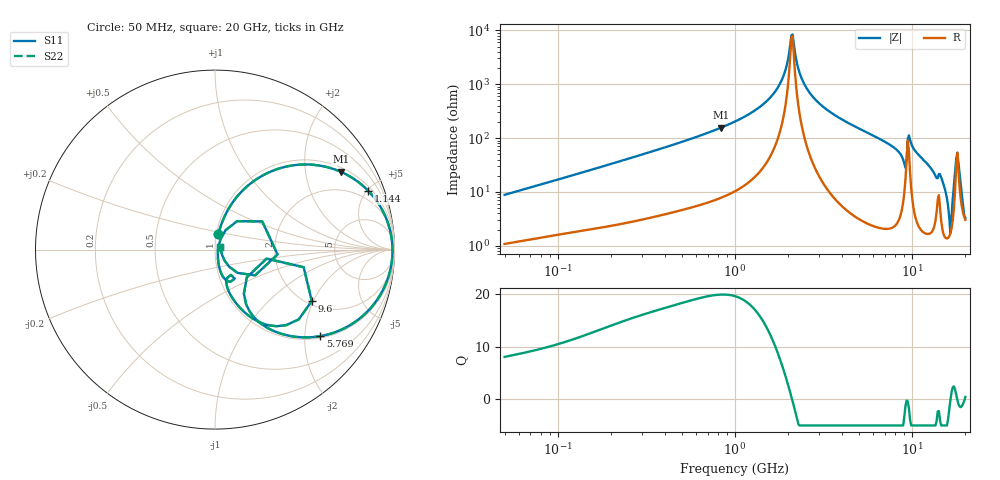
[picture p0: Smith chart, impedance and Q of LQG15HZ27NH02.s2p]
!Murata Part Number: LQG15HZ27NH02
!These Parameters are Measured in Series Mode Connection
!  o--[Z]--o
!Port1  Port2
!  o-------o
!Freq. Start=50[MHz] Stop=20[GHz], 401[Steps]
# Hz S RI R 50
!Freq.(Hz) S11(Real) S11(Imag) S21(Real) S21(Imag) S12(Real) S12(Imag) S22(Real) S22(Imag)
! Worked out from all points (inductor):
!   401 points, 50 MHz to 20 GHz, reference 50 ohm
!   read as one part in series: L = 27.6 nH near 51.52 MHz
!   highest Q = 20 at 835.5 MHz (marker M1), where L = 29.8 nH
!   self-resonance near 2.083 GHz
!   S11 on the Smith chart (normalised r, x): 50 MHz: 1.02, +0.18; 1.144 GHz: 1.27, +5.09; 5.769 GHz: 1.05, -2.39; 9.6 GHz: 2.13, -1.95; 20 GHz: 1.06, +0.03
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5e7  0.0182 0.0854  0.9818 -0.0854  0.9818 -0.0854  0.0182 0.0854
1.364002e8  0.0656 0.2094  0.9344 -0.2094  0.9344 -0.2094  0.0656 0.2094
3.721004e8  0.289 0.425  0.711 -0.425  0.711 -0.425  0.289 0.425
8.354841e8  0.701 0.4335  0.299 -0.4335  0.299 -0.4335  0.701 0.4335
1e9  0.793 0.3806  0.207 -0.3806  0.207 -0.3806  0.793 0.3806
1.144317e9  0.8536 0.3279  0.1464 -0.3279  0.1464 -0.3279  0.8536 0.3279
1.740566e9  0.9743 0.1117  0.0257 -0.1117  0.0257 -0.1117  0.9743 0.1117
1.904239e9  0.9845 0.0589  0.0155 -0.0589  0.0155 -0.0589  0.9845 0.0589
2.083303e9  0.9888 0.00497  0.0112 -0.00497  0.0112 -0.00497  0.9888 0.00497
2.383959e9  0.9836 -0.0768  0.0164 0.0768  0.0164 0.0768  0.9836 -0.0768
2.728004e9  0.9641 -0.1579  0.0359 0.1579  0.0359 0.1579  0.9641 -0.1579
5.769027e9  0.5871 -0.4821  0.4129 0.4821  0.4129 0.4821  0.5871 -0.4821
7.442007e9  0.3714 -0.4697  0.6286 0.4697  0.6286 0.4697  0.3714 -0.4697
8.907419e9  0.1735 -0.3047  0.8265 0.3047  0.8265 0.3047  0.1735 -0.3047
9.600142e9  0.5392 -0.2867  0.4608 0.2867  0.4608 0.2867  0.5392 -0.2867
1.019291e10  0.3044 -0.4228  0.6956 0.4228  0.6956 0.4228  0.3044 -0.4228
1.460232e10  0.0586 -0.1687  0.9414 0.1687  0.9414 0.1687  0.0586 -0.1687
1.621653e10  0.0157 -0.0285  0.9843 0.0285  0.9843 0.0285  0.0157 -0.0285
1.670968e10  0.0215 0.0269  0.9785 -0.0269  0.9785 -0.0269  0.0215 0.0269
1.747767e10  0.1227 0.1583  0.8773 -0.1583  0.8773 -0.1583  0.1227 0.1583
1.800918e10  0.3485 -0.0272  0.6515 0.0272  0.6515 0.0272  0.3485 -0.0272
2e10  0.0297 0.0124  0.9703 -0.0124  0.9703 -0.0124  0.0297 0.0124
